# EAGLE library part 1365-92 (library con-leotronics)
DUAL ROW STRAIGHT HEADER 1364 SERIES. 1.27mm x 1.27mm. Without Fixing Post. SMT Source: http://www.leotronics.co.uk/Conexcon/Data%20Sheets/sec.%20A/1364ing.pdf
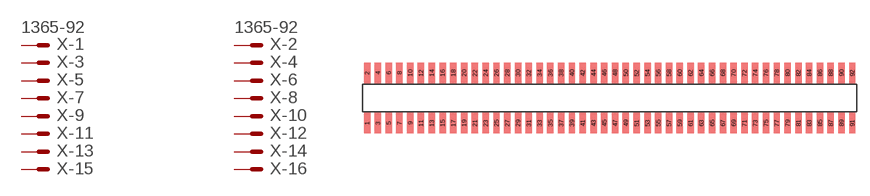
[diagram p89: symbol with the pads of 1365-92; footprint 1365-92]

Designator prefix X; gates -1=MVAL -2=MVAL -3=M -4=M -5=M -6=M -7=M -8=M -9=M -10=M -11=M -12=M -13=M -14=M -15=M -16=M -17=M -18=M -19=M -20=M -21=M -22=M -23=M -24=M -25=M -26=M -27=M -28=M -29=M -30=M -31=M -32=M -33=M -34=M -35=M -36=M -37=M -38=M -39=M -40=M -41=M -42=M -43=M -44=M -45=M -46=M -47=M -48=M -49=M -50=M -51=M -52=M -53=M -54=M -55=M -56=M -57=M -58=M -59=M -60=M -61=M -62=M -63=M -64=M -65=M -66=M -67=M -68=M -69=M -70=M -71=M -72=M -73=M -74=M -75=M -76=M -77=M -78=M -79=M -80=M -81=M -82=M -83=M -84=M -85=M -86=M -87=M -88=M -89=M -90=M -91=M -92=M

## 1365-92 (OC_FARNELL: unknown; OC_NEWARK: unknown)  [1365-92]
1  -1:S  pas
2  -2:S  pas
3  -3:S  pas
4  -4:S  pas
5  -5:S  pas
6  -6:S  pas
7  -7:S  pas
8  -8:S  pas
9  -9:S  pas
10  -10:S  pas
11  -11:S  pas
12  -12:S  pas
13  -13:S  pas
14  -14:S  pas
15  -15:S  pas
16  -16:S  pas
17  -17:S  pas
18  -18:S  pas
19  -19:S  pas
20  -20:S  pas
21  -21:S  pas
22  -22:S  pas
23  -23:S  pas
24  -24:S  pas
25  -25:S  pas
26  -26:S  pas
27  -27:S  pas
28  -28:S  pas
29  -29:S  pas
30  -30:S  pas
31  -31:S  pas
32  -32:S  pas
33  -33:S  pas
34  -34:S  pas
35  -35:S  pas
36  -36:S  pas
37  -37:S  pas
38  -38:S  pas
39  -39:S  pas
40  -40:S  pas
41  -41:S  pas
42  -42:S  pas
43  -43:S  pas
44  -44:S  pas
45  -45:S  pas
46  -46:S  pas
47  -47:S  pas
48  -48:S  pas
49  -49:S  pas
50  -50:S  pas
51  -51:S  pas
52  -52:S  pas
53  -53:S  pas
54  -54:S  pas
55  -55:S  pas
56  -56:S  pas
57  -57:S  pas
58  -58:S  pas
59  -59:S  pas
60  -60:S  pas
61  -61:S  pas
62  -62:S  pas
63  -63:S  pas
64  -64:S  pas
65  -65:S  pas
66  -66:S  pas
67  -67:S  pas
68  -68:S  pas
69  -69:S  pas
70  -70:S  pas
71  -71:S  pas
72  -72:S  pas
73  -73:S  pas
74  -74:S  pas
75  -75:S  pas
76  -76:S  pas
77  -77:S  pas
78  -78:S  pas
79  -79:S  pas
80  -80:S  pas
81  -81:S  pas
82  -82:S  pas
83  -83:S  pas
84  -84:S  pas
85  -85:S  pas
86  -86:S  pas
87  -87:S  pas
88  -88:S  pas
89  -89:S  pas
90  -90:S  pas
91  -91:S  pas
92  -92:S  pas

## Footprint 1365-92 (pad centres in mm)
DUAL ROW STRAIGHT HEADER 1364 SERIES. 1.27mm x 1.27mm. Without Fixing Post. SMT Source: http://www.leotronics.co.uk/Conexcon/Data%20Sheets/sec.%20A/1364ing.pdf
smd 0.76 x 2.4: 1 -28.575,-2.95; 2 -28.575,2.95; 3 -27.305,-2.95; 4 -27.305,2.95; 5 -26.035,-2.95; 6 -26.035,2.95; 7 -24.765,-2.95; 8 -24.765,2.95; 9 -23.495,-2.95; 10 -23.495,2.95; 11 -22.225,-2.95; 12 -22.225,2.95; 13 -20.955,-2.95; 14 -20.955,2.95; 15 -19.685,-2.95; 16 -19.685,2.95; 17 -18.415,-2.95; 18 -18.415,2.95; 19 -17.145,-2.95; 20 -17.145,2.95; 21 -15.875,-2.95; 22 -15.875,2.95; 23 -14.605,-2.95; 24 -14.605,2.95; 25 -13.335,-2.95; 26 -13.335,2.95; 27 -12.065,-2.95; 28 -12.065,2.95; 29 -10.795,-2.95; 30 -10.795,2.95; 31 -9.525,-2.95; 32 -9.525,2.95; 33 -8.255,-2.95; 34 -8.255,2.95; 35 -6.985,-2.95; 36 -6.985,2.95; 37 -5.715,-2.95; 38 -5.715,2.95; 39 -4.445,-2.95; 40 -4.445,2.95; 41 -3.175,-2.95; 42 -3.175,2.95; 43 -1.905,-2.95; 44 -1.905,2.95; 45 -0.635,-2.95; 46 -0.635,2.95; 47 0.635,-2.95; 48 0.635,2.95; 49 1.905,-2.95; 50 1.905,2.95; 51 3.175,-2.95; 52 3.175,2.95; 53 4.445,-2.95; 54 4.445,2.95; 55 5.715,-2.95; 56 5.715,2.95; 57 6.985,-2.95; 58 6.985,2.95; 59 8.255,-2.95; 60 8.255,2.95; 61 9.525,-2.95; 62 9.525,2.95; 63 10.795,-2.95; 64 10.795,2.95; 65 12.065,-2.95; 66 12.065,2.95; 67 13.335,-2.95; 68 13.335,2.95; 69 14.605,-2.95; 70 14.605,2.95; 71 15.875,-2.95; 72 15.875,2.95; 73 17.145,-2.95; 74 17.145,2.95; 75 18.415,-2.95; 76 18.415,2.95; 77 19.685,-2.95; 78 19.685,2.95; 79 20.955,-2.95; 80 20.955,2.95; 81 22.225,-2.95; 82 22.225,2.95; 83 23.495,-2.95; 84 23.495,2.95; 85 24.765,-2.95; 86 24.765,2.95; 87 26.035,-2.95; 88 26.035,2.95; 89 27.305,-2.95; 90 27.305,2.95; 91 28.575,-2.95; 92 28.575,2.95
